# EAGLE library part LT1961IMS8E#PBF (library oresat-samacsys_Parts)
Step-Up Switching Regulator Source: Datasheet
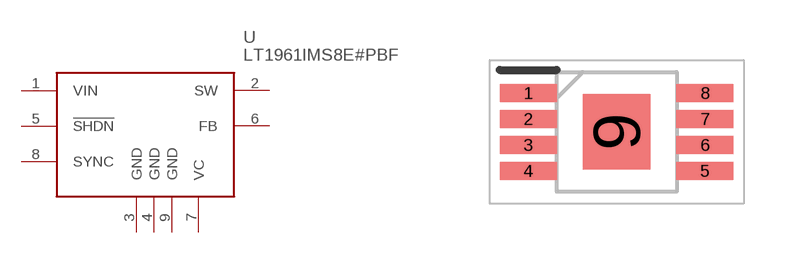
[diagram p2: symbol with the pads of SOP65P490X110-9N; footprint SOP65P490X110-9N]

Designator prefix U

## LT1961IMS8E#PBF (DESCRIPTION: Step-Up Switching Regulator; HEIGHT: 1.1mm; MANUFACTURER_NAME: Linear Technology; MPN: LT1961IMS8E#PBF; VALUE: LT1961IMS8E)  [SOP65P490X110-9N]
1  VIN  pwr
2  SW
3  GND  pwr
4  GND  pwr
5  !SHDN
6  FB
7  VC
8  SYNC
9  GND  pwr

## Footprint SOP65P490X110-9N (pad centres in mm)
MS8E(MSOP)
smd 1.425 x 0.45: 1 -2.212,0.975; 2 -2.212,0.325; 3 -2.212,-0.325; 4 -2.212,-0.975; 5 2.212,-0.975; 6 2.212,-0.325; 7 2.212,0.325; 8 2.212,0.975
smd 1.68 x 1.88: 9 0,0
